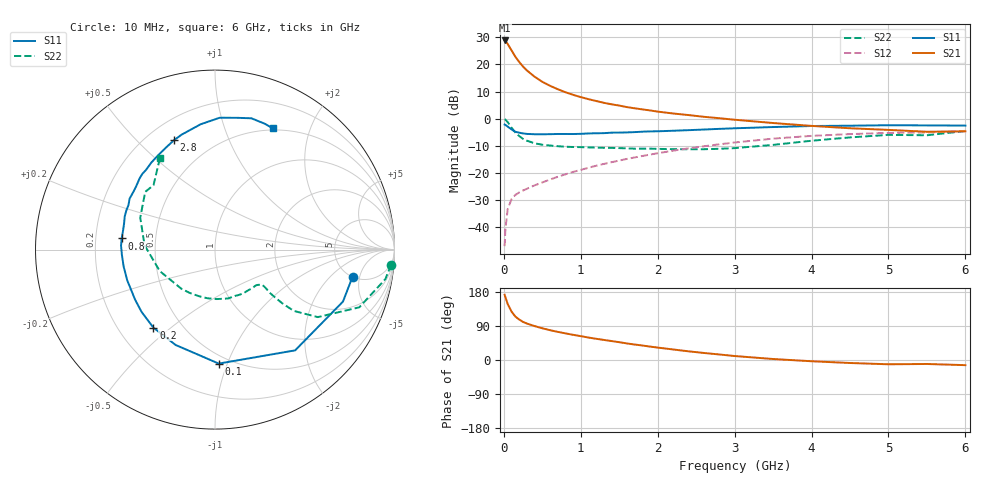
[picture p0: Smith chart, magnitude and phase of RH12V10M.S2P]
! SIEMENS Small Signal Semiconductors
! BFR106
! Si NPN RF Bipolar Junction Transistor in SOT23
! VCE = 12 V  IC = 10 mA
! Common Emitter S-Parameters:  August  1996
# GHz  S  MA  R  50
!  f  S11  S21  S12  S22
! GHz  MAG  ANG  MAG  ANG  MAG  ANG  MAG  ANG
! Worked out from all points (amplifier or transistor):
!   36 points, 10 MHz to 6 GHz, reference 50 ohm
!   highest |S21| = 28.8 dB at 10 MHz (marker M1)
!   |S21| within 3 dB of that: start of sweep to 86.16 MHz
!   unconditionally stable (mu >= 1): 491.9 MHz to 1.898 GHz; 5.376 GHz to end of sweep
!   at 250 MHz: K = 0.70, MSG = 22.8 dB, |S12| = -26.4 dB
!   at 1.4 GHz: K = 1.08, MAG = 8.9 dB, |S12| = -16.0 dB
!   at 6 GHz: K = 1.01, MAG = -0.5 dB, |S12| = -4.5 dB
!   S11 on the Smith chart (normalised r, x): 10 MHz: 5.02, -3.91; 100 MHz: 0.44, -0.93; 200 MHz: 0.35, -0.44; 800 MHz: 0.31, +0.05; 2.8 GHz: 0.31, +0.65; 6 GHz: 0.48, +1.47
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0.01  0.7811 -11.2  27.65 172.1  0.0045 84.8  0.9847 -4.9
0.02  0.7696 -22.1  27.12 166.0  0.0091 79.2  0.9638 -9.8
0.05  0.7173 -51.5  23.8 147.7  0.0216 66.5  0.8657 -21.8
0.1  0.6354 -88.1  18.16 127.8  0.0331 54.5  0.6852 -33.3
0.15  0.575 -112.4  13.84 114.5  0.0396 48.5  0.5559 -37.9
0.2  0.5539 -128.3  11.1 106.8  0.044 48.5  0.48 -38.6
0.25  0.5363 -139.8  9.122 100.4  0.0477 47.9  0.4256 -38.5
0.3  0.5254 -147.9  7.744 96.2  0.0513 49.8  0.3935 -38.3
0.4  0.5181 -160.8  5.938 89.5  0.0593 52.8  0.3532 -37.1
0.5  0.5176 -169.4  4.789 83.7  0.0671 55.9  0.3319 -36.7
0.6  0.5195 -176.7  4.046 78.7  0.0759 58.0  0.3211 -37.5
0.8  0.5237 173.2  3.08 70.3  0.0947 61.0  0.305 -40.4
0.9  0.523 168.4  2.755 66.5  0.1049 62.3  0.3016 -42.0
1.1  0.536 159.8  2.295 59.3  0.1251 63.4  0.2966 -47.4
1.3  0.5422 152.8  1.966 53.0  0.1472 63.7  0.2915 -52.9
1.6  0.5599 142.9  1.638 43.7  0.1819 63.0  0.2848 -63.1
2.2  0.6013 126.0  1.25 27.8  0.258 58.4  0.2758 -87.8
2.8  0.6506 110.6  1.023 14.6  0.3379 50.8  0.2794 -120.0
3.5  0.703 96.5  0.834 2.6  0.4302 39.9  0.3301 -158.7
4.5  0.7443 80.6  0.668 -7.9  0.5215 22.2  0.4531 156.8
5.5  0.754 68.4  0.576 -10.5  0.5571 9.7  0.496 133.7
6  0.7482 64.6  0.586 -13.6  0.5972 1.7  0.5945 121.1
